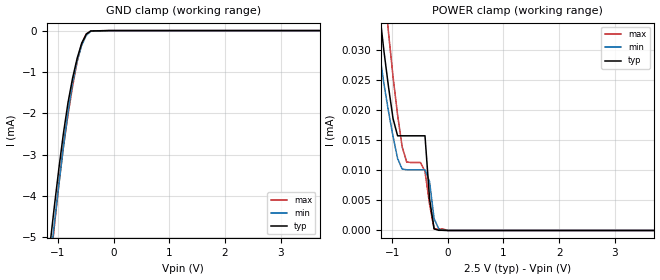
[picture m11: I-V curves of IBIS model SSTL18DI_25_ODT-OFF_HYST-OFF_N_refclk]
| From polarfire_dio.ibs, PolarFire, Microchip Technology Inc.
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|   Model SSTL18DI_25_ODT-OFF_HYST-OFF_N_refclk
[Model]   SSTL18DI_25_ODT-OFF_HYST-OFF_N_refclk
Model_type   Input
Vinl =   0.775
Vinh =   1.025
|   typ   min   max
C_comp   2.671e-12   2.671e-12   2.761e-12
[Temperature Range]  25C   100C   -40C
[Voltage Range]  2.5   2.375   2.625
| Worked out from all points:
|   GND clamp passes 1 mA (typ) near -0.71 V on its own axis
[GND Clamp]
| Voltage   I(typ)   I(min)   I(max)
-2.5V     -29.41mA   -28.65mA   -32.17mA
-1.148V   -5.231mA   -5.664mA   -5.827mA
-1.066V   -4.254mA   -4.675mA   -4.737mA
-984.4mV  -3.331mA   -3.717mA   -3.705mA
-902.3mV  -2.478mA   -2.807mA   -2.8mA
-820.3mV  -1.738mA   -1.973mA   -2.031mA
-738.3mV  -1.148mA   -1.262mA   -1.341mA
-656.2mV  -667.7uA   -728.5uA   -750.4uA
-574.2mV  -304.1uA   -352.5uA   -314.1uA
-492.2mV  -84.35uA   -112uA     -81.68uA
-410.2mV  -8.907uA   -16.99uA   -8.147uA
5V        0A         0A         0A
[POWER Clamp]
| Voltage   I(typ)   I(min)   I(max)
-2.5V     172.7uA    122.1uA    221.5uA
-1.312V   43.36uA    35.03uA    58.78uA
-1.148V   29.9uA     24.47uA    41uA
-1.066V   23.96uA    19.84uA    33.02uA
-902.3mV  15.76uA    11.98uA    19.22uA
-820.3mV  15.76uA    10.22uA    13.92uA
-738.3mV  15.76uA    10.1uA     11.38uA
-410.2mV  15.76uA    10.1uA     9.823uA
-328.1mV  5.279uA    8.13uA     4.402uA
-246.1mV  271.7nA    1.95uA     233.8nA
-82.03mV  29.34nA    23.29nA    233.8nA
5V        0A         0A         0A
